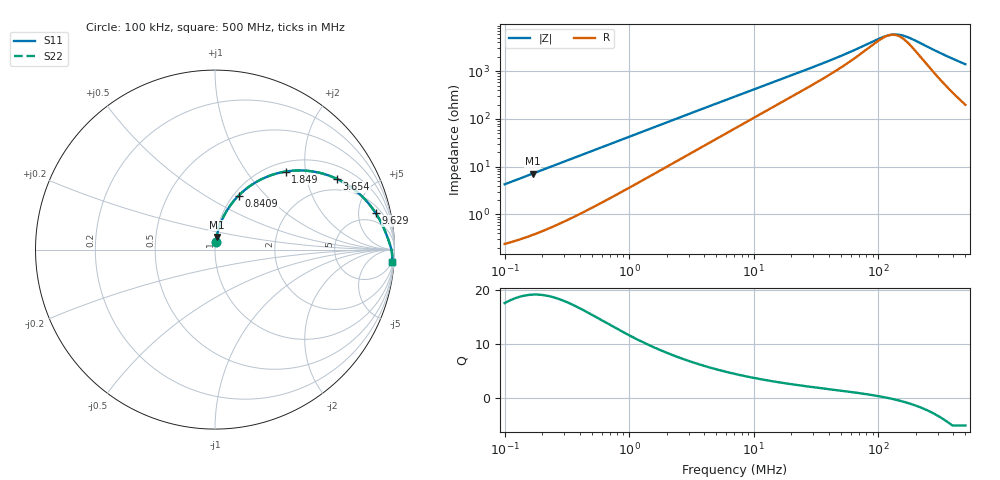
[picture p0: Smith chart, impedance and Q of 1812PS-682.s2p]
# MHz S MA R 50
!Freq  MagS11  AngS11  MagS21  AngS21  MagS12  AngS12  MagS22  AngS22
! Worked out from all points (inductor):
!   801 points, 100 kHz to 500 MHz, reference 50 ohm
!   read as one part in series: L = 6.79 uH near 104.4 kHz
!   highest Q = 19.2 at 168.5 kHz (marker M1), where L = 6.79 uH
!   self-resonance near 124.7 MHz
!   S11 on the Smith chart (normalised r, x): 100 kHz: 1.00, +0.09; 840.9 kHz: 1.06, +0.71; 1.849 MHz: 1.18, +1.56; 3.654 MHz: 1.48, +3.05; 9.629 MHz: 3.00, +7.75; 500 MHz: 5, -28
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0.1  0.04261 84.3  0.9967 -2.4  0.9967 -2.4  0.04261 84.3
0.1684853  0.07152 82.9  0.9937 -4.1  0.9937 -4.1  0.07152 82.9
0.416464  0.1731 76.6  0.9745 -10.0  0.9745 -10.0  0.1731 76.6
0.6045155  0.2455 71.9  0.9526 -14.2  0.9526 -14.2  0.2455 71.9
0.8408964  0.329 66.3  0.9187 -19.1  0.9187 -19.1  0.329 66.3
1.194882  0.437 58.9  0.86 -25.8  0.86 -25.8  0.437 58.9
1.716055  0.5605 49.9  0.7693 -33.9  0.7693 -33.9  0.5605 49.9
1.848831  0.5859 47.9  0.7468 -35.6  0.7468 -35.6  0.5859 47.9
2.571771  0.6923 39.1  0.6358 -43.3  0.6358 -43.3  0.6923 39.1
3.654389  0.7848 30.2  0.5089 -50.8  0.5089 -50.8  0.7848 30.2
5.029516  0.8462 23.2  0.4003 -56.3  0.4003 -56.3  0.8462 23.2
7.071068  0.8909 17.1  0.3013 -60.5  0.3013 -60.5  0.8909 17.1
9.628811  0.9179 12.8  0.2293 -62.7  0.2293 -62.7  0.9179 12.8
16.39677  0.946 7.6  0.1403 -63.6  0.1403 -63.6  0.946 7.6
29.44845  0.9631 4.2  0.08008 -60.5  0.08008 -60.5  0.9631 4.2
54.60568  0.974 1.9  0.04231 -51.1  0.04231 -51.1  0.974 1.9
103.4333  0.9813 0.4  0.01993 -20.0  0.01993 -20.0  0.9813 0.4
121.3434  0.9827 0.1  0.01734 -3.3  0.01734 -3.3  0.9827 0.1
142.3547  0.9839 -0.3  0.01677 16.8  0.01677 16.8  0.9839 -0.3
168.7918  0.9851 -0.7  0.01868 36.9  0.01868 36.9  0.9851 -0.7
344.461  0.988 -2.6  0.04591 73.6  0.04591 73.6  0.988 -2.6
500  0.9876 -4.0  0.07051 77.9  0.07051 77.9  0.9876 -4.0
